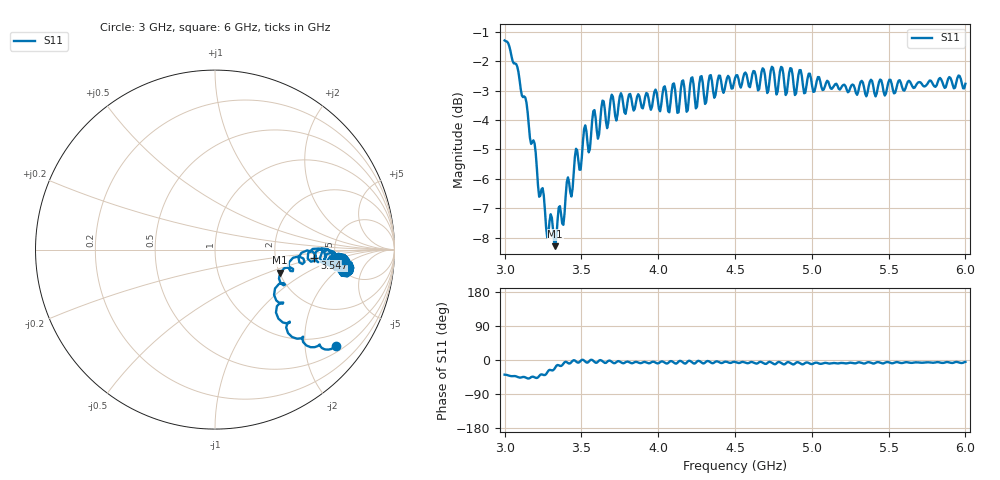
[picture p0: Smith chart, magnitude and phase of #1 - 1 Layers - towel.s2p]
!  02/07/2025  16:22:13
! Ref Plane: 0.000 mm
# MHZ S MA R  50
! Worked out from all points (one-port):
!   401 points, 3 GHz to 6 GHz, reference 50 ohm
!   lowest |S11| = -8.3 dB at 3.33 GHz (marker M1), VSWR 2.25, Z = 101 - j30.5 ohm
!   |S11| at or under -10 dB: nowhere
!   S11 on the Smith chart (normalised r, x): 3 GHz: 0.65, -2.71; 3.547 GHz: 3.44, -0.45; 6 GHz: 5.90, -1.56
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3000  0.8611 -38.6
3090  0.7611 -45.6
3217.5  0.4879 -45.9
3330  0.385 -19.6
3375  0.4208 -13.8
3450  0.5133 -0.5
3547.5  0.5558 -4.7
3577.5  0.6531 -2.1
3750  0.6923 -4.1
4065  0.6525 -7.8
4095  0.7257 -4.8
4125  0.6487 -7.5
4155  0.7343 -4.5
4185  0.6515 -7.2
4215  0.7434 -4.4
4245  0.6601 -7.2
4275  0.7472 -4.5
4305  0.6716 -6.9
4500  0.7428 -5.1
4725  0.7376 -4.8
4755  0.7545 -10.9
4785  0.7349 -5.0
4815  0.7546 -11.3
4845  0.7306 -5.3
4875  0.7523 -11.4
5250  0.7148 -7.1
5625  0.7328 -6.1
6000  0.7269 -4.9
